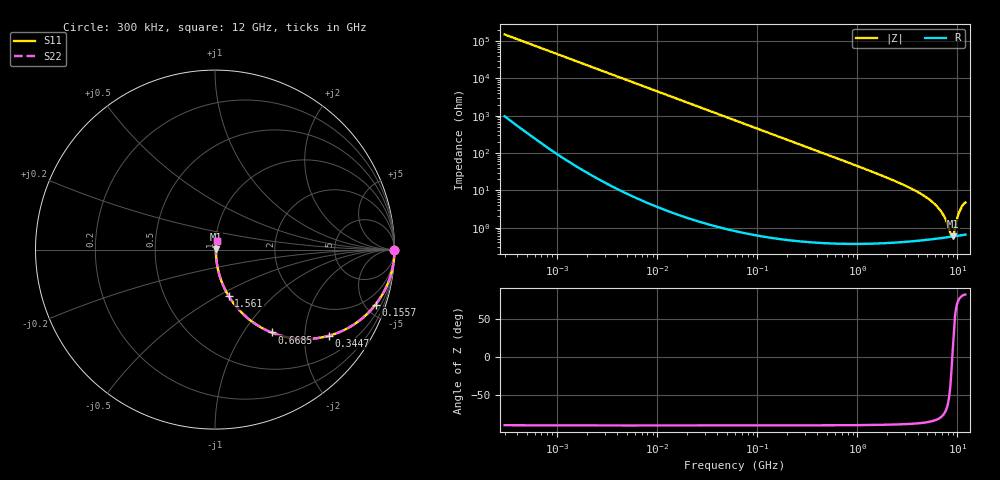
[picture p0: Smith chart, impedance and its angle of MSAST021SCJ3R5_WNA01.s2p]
! MSAST021SCJ3R5_WNA01  S-PARAMETER MODEL  ( General Type )
! Model Generated by TAIYO YUDEN Corporation (http://www.ty-top.com)
! Version 2.0
! TAIYO YUDEN Control No. 181101
! Copyright(c) 2015 TAIYO YUDEN CO.,LTD. All Rights Reserved.
! Product Description (link to TY-COMPAS)
! https://ds.yuden.co.jp/TYCOMPAS/or/detail?pn=MSAST021SCJ3R5BWNA01&u=M
! Products Name : Multilayer Ceramic Capacitors
! Characteristics :
!  Capacitance : 3.5 pF , Rated Voltage : 25V , TCC : CJ / C0J
!  Case Size : 0.25 x 0.125 / 0.0098 x 0.0049 [mm/inch] , Thickness : 0.125 / 0.0049 [mm/inch]
!  (Conditions: Temperature = 25 degC , DC Bias Current/Voltage = 0A / 0V)
! External Node Assignments :
!  1  o---| |---o  2
! GND o---------o GND
! Frequency Range : 0.3MHz  -  12000MHz  [ 401 STEP ]
# MHz S RI R 50
! Freq[MHz].  S11 Real  S11 Imag  S21 Real  S21 Imag  S12 Real  S12 Imag  S22 Real  S22 Imag
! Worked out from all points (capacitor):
!   401 points, 300 kHz to 12 GHz, reference 50 ohm
!   read as one part in series: C = 3.5 pF near 316.3 kHz
!   lowest |Z| = 583 mohm at 8.967 GHz (marker M1)
!   series resonance near 8.881 GHz, so ESL is about 92 pH
!   S11 on the Smith chart (normalised r, x): 300 kHz: open; 155.7 MHz: 1.01, -5.84; 344.7 MHz: 1.01, -2.63; 668.5 MHz: 1.01, -1.35; 1.561 GHz: 1.01, -0.56; 12 GHz: 1.01, +0.09
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0.3  1 -0.00066  4.66e-06 0.00066  4.66e-06 0.00066  1 -0.00066
1.769972  1 -0.00389  2.06e-05 0.00389  2.06e-05 0.00389  1 -0.00389
10.44266  0.9995 -0.023  0.000545 0.023  0.000545 0.023  0.9995 -0.023
60  0.9828 -0.1297  0.0172 0.1297  0.0172 0.1297  0.9828 -0.1297
155.7172  0.8946 -0.3062  0.1054 0.3062  0.1054 0.3062  0.8946 -0.3062
231.6935  0.7931 -0.4039  0.2069 0.4039  0.2069 0.4039  0.7931 -0.4039
344.7396  0.6339 -0.4802  0.3661 0.4802  0.3661 0.4802  0.6339 -0.4802
353.9943  0.6215 -0.4834  0.3785 0.4834  0.3785 0.4834  0.6215 -0.4834
668.5285  0.3148 -0.4617  0.6852 0.4617  0.6852 0.4617  0.3148 -0.4617
1021.415  0.1638 -0.366  0.8362 0.366  0.8362 0.366  0.1638 -0.366
1560.575  0.0768 -0.2597  0.9232 0.2597  0.9232 0.2597  0.0768 -0.2597
2088.533  0.044 -0.1958  0.956 0.1958  0.956 0.1958  0.044 -0.1958
3740.715  0.0141 -0.0981  0.9859 0.0981  0.9859 0.0981  0.0141 -0.0981
5565.855  0.00726 -0.0489  0.9927 0.0489  0.9927 0.0489  0.00726 -0.0489
6879.757  0.00588 -0.026  0.9941 0.026  0.9941 0.026  0.00588 -0.026
7648.807  0.00563 -0.0151  0.9944 0.0151  0.9944 0.0151  0.00563 -0.0151
8503.825  0.00563 -0.00426  0.9944 0.00426  0.9944 0.00426  0.00563 -0.00426
8966.534  0.00573 0.000906  0.9943 -0.000906  0.9943 -0.000906  0.00573 0.000906
9207.246  0.0058 0.00344  0.9942 -0.00344  0.9942 -0.00344  0.0058 0.00344
10511.28  0.00682 0.0267  0.9932 -0.0267  0.9932 -0.0267  0.00682 0.0267
11380.75  0.00795 0.0404  0.9921 -0.0404  0.9921 -0.0404  0.00795 0.0404
12000  0.00855 0.0458  0.9914 -0.0458  0.9914 -0.0458  0.00855 0.0458
